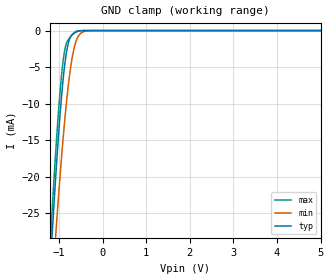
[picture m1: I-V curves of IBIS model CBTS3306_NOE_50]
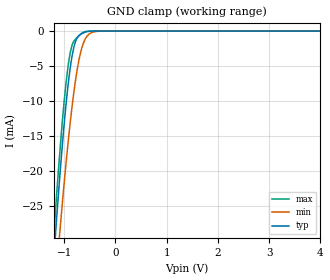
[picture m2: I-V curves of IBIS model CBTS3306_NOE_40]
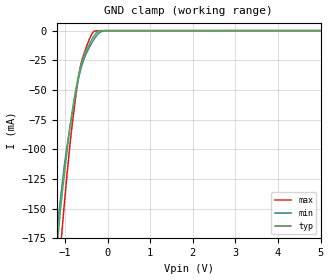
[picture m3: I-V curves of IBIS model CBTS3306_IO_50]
| TEXAS INSTRUMENTS INCORPORATED
| Standard Linear and Logic Group
| IBIS Model of SN74CBTS3306
| DUAL FET BUS SWITCH WITH SCHOTTKY DIODE CLAMPING
| This file contains package information for the following:
|  SOIC 8-pin (D) package as [Component] CBTS3306_D
|  TSSOP 8-pin (PW) package as [Component] CBTS3306_PW
| This device can be powered at the following Vccs:
|  5 volt Vcc
|  4 volt Vcc
| This file provides unique models under the [Model Selector] for each Vcc.
| For operation at a specific Vcc, select the appropriate model after each
| [Model Selector] keyword.
[IBIS Ver]   3.2
[Comment char]  |_char
[File Name]   sn74cbts3306.ibs
[File Rev]   1.1 | e_die
[Date]   July 10, 2002
[Source]   Data created from TI-SPICE simulations at TI-SLL.
[Notes]   The following is an IBIS list for the SN74CBTS3306.
   Please contact sllibis@ti.com with questions and
   comments concerning SLL IBIS models.
   This IBIS model is created from a BA (back annotated netlist).
   IBISCHK3.2.8 Cannot handle model selector keyword
   for series pin mapping. Please remove comment
   charecters from specific models in the
   series pin mapping.
[Disclaimer] Property of Texas Instruments Incorporated. Unauthorized
   reproduction and/or distribution is strictly prohibited.
   This product is protected under copyright law.
   Created 2002, (C) Copyright 2002, Texas Instruments
   Incorporated, All Rights Reserved
   UNLESS THERE IS A SIGNED, WRITTEN AGREEMENT TO THE
   CONTRARY, TEXAS INSTRUMENTS (TI) IS PROVIDING THE IBIS
   MODELS  AND WITHOUT ANY WARRANTY, EXPRESSED OR
   IMPLIED. TI assumes no liability for:
   1) the accuracy of the IBIS models provided to your
   company;
   2) the proper functioning of these IBIS Models in your
   design or for any resulting applications; or
   3) infringement of patents, copyrights or intellectual
   property rights resulting from your use of these IBIS
   models.
   TI provides IBIS Models as a service to our customers.
   You and your company shall not distribute, sell or give
   these models to anyone else without prior written
   permission from TI.
   TI reserves the right to make changes to our products or
   to discontinue any semiconductor product or service
   without notice, and advises our customers to obtain the
   latest version of relevant information to verify, before
   placing orders, that the information being relied on is
   current.
   Please be aware that your receipt and use of the IBIS
   information provided shall serve as acceptance of these
   terms and conditions. If you do not accept these terms,
   you should return or destroy the IBIS models and any
   other accompanying information immediately.
| Component CBTS3306_D 8-pin SOIC
[Component]   CBTS3306_D
[Manufacturer]   Texas Instruments, Inc.
[Package]
|   typ   min   max
R_pkg   2.600e-02   1.700e-02   3.500e-02
L_pkg   2.637e-09   2.180e-09   3.093e-09
C_pkg   2.690e-13   2.240e-13   3.130e-13
[Pin]   signal_name   model_name   R_pin   L_pin   C_pin
1   1NOE   CBTS3306_NOE   3.500e-02   3.093e-09   3.130e-13
2   1A   CBTS3306_IO   1.700e-02   2.180e-09   2.240e-13
3   1B   CBTS3306_IO   1.700e-02   2.180e-09   2.240e-13
4   GND   GND   3.500e-02   3.093e-09   3.130e-13
5   2A   CBTS3306_IO   3.500e-02   3.093e-09   3.130e-13
6   2B   CBTS3306_IO   1.700e-02   2.180e-09   2.240e-13
7   2NOE   CBTS3306_NOE   1.700e-02   2.180e-09   2.240e-13
8   VCC   POWER   3.500e-02   3.093e-09   3.130e-13
| Component CBTS3306_PW 8-pin TSSOP
[Component]   CBTS3306_PW
[Manufacturer]   Texas Instruments, Inc.
[Package]
|   typ   min   max
R_pkg   0.040   0.034   0.046
L_pkg   2.625nH   2.419nH   2.861nH
C_pkg   0.304pF   0.286pF   0.321pF
[Pin]   signal_name   model_name   R_pin   L_pin   C_pin
1   1NOE   CBTS3306_NOE   0.046   2.861nH   0.321pF
2   1A   CBTS3306_IO   0.037   2.437nH   0.286pF
3   1B   CBTS3306_IO   0.034   2.419nH   0.286pF
4   GND   GND   0.043   2.784nH   0.321pF
5   2A   CBTS3306_IO   0.043   2.784nH   0.321pF
6   2B   CBTS3306_IO   0.035   2.420nH   0.286pF
7   2NOE   CBTS3306_NOE   0.037   2.437nH   0.286pF
8   VCC   POWER   0.046   2.860nH   0.321pF
[Series Switch Groups]
| Function Group States
On  1 /   | 1A->1B 1NOE LOW
   | 2A->2B 2NOE LOW
[Series Pin Mapping]   pin_2   model_name   function_table_group
2   3   CBTS3306_IO_50_S   1
|2   3   CBTS3306_IO_40_S   1
5   6   CBTS3306_IO_50_S   1
|5   6   CBTS3306_IO_40_S   1
| Model CBTS3306_NOE
[Model Selector]   CBTS3306_NOE
CBTS3306_NOE_50   5 volt Vcc
CBTS3306_NOE_40   4 volt Vcc
| Model CBTS3306_IO
[Model Selector]   CBTS3306_IO
CBTS3306_IO_50   5 volt Vcc
CBTS3306_IO_40   4 volt Vcc
| Model CBTS3306_IO_S
[Model Selector]   CBTS3306_IO_S
CBTS3306_IO_50_S   5 volt Vcc
CBTS3306_IO_40_S   4 volt Vcc
[Model]   CBTS3306_IO_50_S
Model_type  Series_switch
| variable   typ   min   max
C_comp   0   0   0
[Temperature Range]   40   100   -40
| Ambient temperature   25   85   -40
[Voltage range]   5   4.5   5.5
[On]
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[Off]
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[Model]   CBTS3306_IO_40_S
Model_type  Series_switch
| variable   typ   min   max
C_comp   0   0   0
[Temperature Range]   40   100   -40
| Ambient temperature   25   85   -40
[Voltage range]   4   4   4
[On]
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[Off]
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| Models and submodels in the file (6): CBTS3306_NOE_50 (Input), CBTS3306_NOE_40 (Input), CBTS3306_IO_50_S (Series_switch), CBTS3306_IO_50 (Terminator), CBTS3306_IO_40_S (Series_switch), CBTS3306_IO_40 (Terminator)
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[Model]   CBTS3306_NOE_50
Model_type  Input
Vinl = 0.8
Vinh = 3.575
| variable   typ   min   max
C_comp   5pF   NA   NA
[Temperature Range]   40   100   -40
| Ambient temperature   25   85   -40
[Voltage range]   5   4.5   5.5
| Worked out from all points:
|   GND clamp passes 1 mA (typ) near -0.75 V on its own axis
[GND Clamp]
| CBTS3306_NOE_50
|   Voltage   I(typ)   I(min)   I(max)
-5V       -499.3mA   -428.8mA   -513.4mA
-1.185V   -30.81mA   -37.71mA   -27.5mA
-1.155V   -27.73mA   -35mA      -24.37mA
-1.06V    -18.58mA   -26.73mA   -15.19mA
-975mV    -11.46mA   -19.88mA   -8.326mA
-900mV    -6.364mA   -14.4mA    -3.922mA
-845mV    -3.604mA   -10.82mA   -2.038mA
-780mV    -1.57mA    -7.182mA   -1.182mA
-695mV    -558.9uA   -3.611mA   -543.9uA
-605mV    -200.3uA   -1.406mA   -101.8uA
-300mV    -29.91nA   -10.05uA   -1.516nA
5V        5.273nA    13.66nA    5.224nA
[Model]   CBTS3306_NOE_40
Model_type  Input
Vinl = 0.8
Vinh = 2.6
| variable   typ   min   max
C_comp   5pF   NA   NA
[Temperature Range]   40   100   -40
| Ambient temperature   25   85   -40
[Voltage range]   4   4   4
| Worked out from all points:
|   GND clamp passes 1 mA (typ) near -0.75 V on its own axis
[GND Clamp]
| CBTS3306_NOE_40
|   Voltage   I(typ)   I(min)   I(max)
-4V       -375.2mA   -325.1mA   -384.7mA
-1.195V   -31.85mA   -38.63mA   -28.56mA
-1.175V   -29.77mA   -36.81mA   -26.44mA
-1.155V   -27.73mA   -35mA      -24.37mA
-1.075V   -19.96mA   -28mA      -16.55mA
-985mV    -12.23mA   -20.65mA   -9.043mA
-905mV    -6.65mA    -14.74mA   -4.153mA
-780mV    -1.57mA    -7.182mA   -1.182mA
-630mV    -281.3uA   -1.867mA   -182uA
-500mV    -26.89uA   -368.6uA   -5.52uA
-310mV    -46.05nA   -12.73uA   -1.776nA
4V        4.259nA    10.47nA    4.19nA
[Model]   CBTS3306_IO_50
Model_type  Terminator
| variable   typ   min   max
C_comp   6pF   NA   NA
| C_tri-state   15.64pF   7.44pF   48.24pF
[Temperature Range]   40   100   -40
| Ambient temperature   25   85   -40
[Voltage range]   5   4.5   5.5
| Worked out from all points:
|   GND clamp passes 1 mA (typ) near -0.24 V on its own axis
[GND Clamp]
| CBTS3306_IO_50
|   Voltage   I(typ)   I(min)   I(max)
-5V       -3.028A    -3.008A    -2.904A
-1.245V   -206.1mA   -186.4mA   -245mA
-1.18V    -179.6mA   -165.1mA   -215.7mA
-1.11V    -151.6mA   -142.6mA   -185.1mA
-1.06V    -135mA     -126.9mA   -163.9mA
-860mV    -75.65mA   -75.23mA   -88.04mA
-680mV    -37.59mA   -39.82mA   -38.3mA
-555mV    -21.13mA   -23.86mA   -19.45mA
-320mV    -4.302mA   -7.31mA    -632.9uA
-185mV    -217.7uA   -1.458mA   -1.815uA
-45mV     -1.696uA   -35.04uA   -3.318nA
5V        4.324uA    59.27uA    62.03nA
